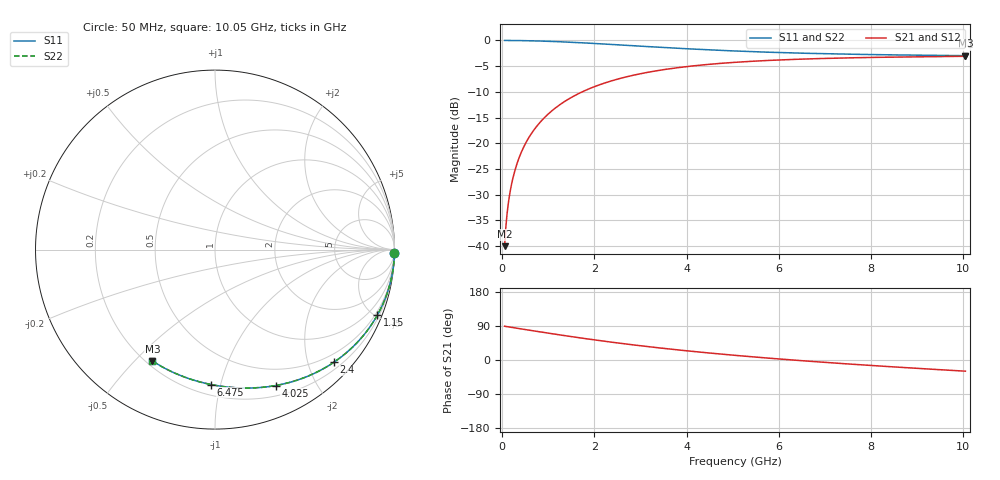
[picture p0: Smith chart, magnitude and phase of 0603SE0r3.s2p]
! AVX Thin Film Operation		Date: August 2001
! Description: Accu-P® Series, Thin Film, SMD, RF Capacitor
! Part Number: 06035J0R3ABT
! 50 MHz  -  10.05 GHz
! Serial Measurements
# mhz S db R 50
!	S11		S21		S12		S22
!	dB	Phase	dB	Phase	dB	Phase	dB	Phase
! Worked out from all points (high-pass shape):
!   401 points, 50 MHz to 10.05 GHz, reference 50 ohm
!   highest |S21| = -3.08 dB at 10.05 GHz (marker M1); lowest = -40.0 dB at 50 MHz (marker M2)
!   |S21| within 3 dB of the highest: 3.229 GHz to end of sweep
!   lowest |S11| = -3.0 dB at 10.05 GHz (marker M3), VSWR 5.93, Z = 11.2 - j28.1 ohm
!   |S11| at or under -10 dB: nowhere
!   |S22| runs from -3.0 to 0.0 dB; largest |S21 - S12| = 0
!   S11 on the Smith chart (normalised r, x): 50 MHz: open; 1.15 GHz: 0.34, -5.13; 2.4 GHz: 0.33, -2.48; 4.025 GHz: 0.31, -1.50; 6.475 GHz: 0.27, -0.94; 10.05 GHz: 0.22, -0.56
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50  -0.00 -1.0  -40.04 89.1  -40.04 89.1  -0.00 -1.0
75  -0.00 -1.5  -36.52 88.6  -36.52 88.6  -0.00 -1.5
125  -0.00 -2.4  -32.09 87.6  -32.09 87.6  -0.00 -2.4
150  -0.00 -2.9  -30.51 87.1  -30.51 87.1  -0.00 -2.9
200  -0.01 -3.9  -28.01 86.1  -28.01 86.1  -0.01 -3.9
275  -0.01 -5.4  -25.26 84.7  -25.26 84.7  -0.01 -5.3
375  -0.02 -7.3  -22.58 82.7  -22.58 82.7  -0.02 -7.3
525  -0.05 -10.2  -19.69 79.8  -19.69 79.8  -0.05 -10.2
700  -0.08 -13.5  -17.25 76.5  -17.25 76.5  -0.08 -13.5
900  -0.14 -17.3  -15.16 72.7  -15.16 72.7  -0.14 -17.3
1150  -0.21 -22.0  -13.16 68.0  -13.16 68.0  -0.22 -22.0
1425  -0.32 -27.0  -11.47 63.0  -11.47 63.0  -0.32 -27.0
1725  -0.45 -32.2  -10.04 57.7  -10.04 57.7  -0.45 -32.2
2400  -0.79 -43.4  -7.79 46.6  -7.79 46.6  -0.79 -43.4
2875  -1.04 -50.6  -6.71 39.4  -6.71 39.4  -1.04 -50.5
3400  -1.32 -57.9  -5.83 32.0  -5.83 32.0  -1.32 -57.9
4025  -1.62 -66.0  -5.07 24.0  -5.07 24.0  -1.62 -65.9
5050  -2.05 -77.7  -4.26 12.3  -4.26 12.3  -2.05 -77.6
6475  -2.47 -91.6  -3.64 -1.6  -3.64 -1.6  -2.47 -91.5
6725  -2.53 -93.8  -3.57 -3.8  -3.57 -3.8  -2.53 -93.7
8400  -2.80 -107.4  -3.25 -17.5  -3.25 -17.5  -2.80 -107.4
10050  -2.96 -119.4  -3.08 -29.5  -3.08 -29.5  -2.96 -119.3
